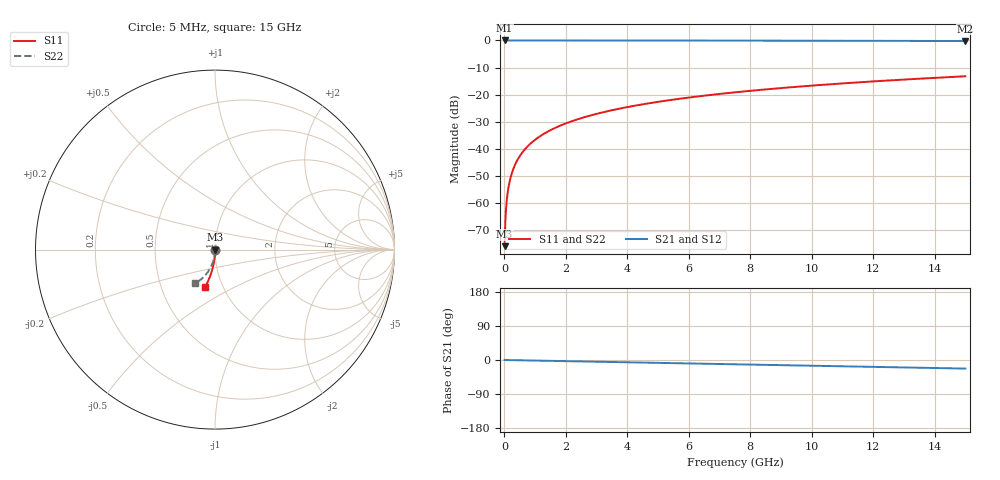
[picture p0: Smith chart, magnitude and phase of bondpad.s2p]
! Created Wed Jan 20 14:36:55 2021
# hz S ma R 50
! 2 Port Network Data from SP1.SP block
! freq  magS11  angS11  magS21  angS21  magS12  angS12  magS22  angS22
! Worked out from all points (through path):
!   3000 points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, 5 MHz to 15 GHz, reference 50 ohm
!   highest |S21| = 0.00 dB at 5 MHz (marker M1); lowest = -0.2 dB at 15 GHz (marker M2)
!   group delay of S21, straight-line fit = 4.19 ps
!   lowest |S11| = -75.9 dB at 5 MHz (marker M3), VSWR 1.00, Z = 50 - j0.00742 ohm
!   |S11| at or under -10 dB: start of sweep to end of sweep
!   |S22| runs from -75.9 to -13.2 dB; largest |S21 - S12| = 0
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5000000  0.0001606 -27.5  0.9999 -0.0  0.9999 -0.0  0.0001606 -27.5
4e7  0.0006096 -76.5  0.9999 -0.1  0.9999 -0.1  0.0006093 -76.5
8.5e7  0.001267 -83.6  0.9999 -0.1  0.9999 -0.1  0.001266 -83.7
1e8  0.001488 -84.6  0.9999 -0.2  0.9999 -0.2  0.001487 -84.7
1.3e8  0.00193 -85.9  0.9998 -0.2  0.9998 -0.2  0.001929 -86.0
1.7e8  0.00252 -86.9  0.9998 -0.3  0.9998 -0.3  0.002519 -87.1
2.3e8  0.003407 -87.8  0.9998 -0.3  0.9998 -0.3  0.003405 -88.0
3.1e8  0.004589 -88.5  0.9998 -0.5  0.9998 -0.5  0.004586 -88.8
4.1e8  0.006067 -89.0  0.9998 -0.6  0.9998 -0.6  0.006063 -89.4
5.25e8  0.007766 -89.5  0.9998 -0.8  0.9998 -0.8  0.007761 -90.0
6.7e8  0.009909 -89.8  0.9998 -1.0  0.9998 -1.0  0.009903 -90.5
8.4e8  0.01242 -90.2  0.9997 -1.3  0.9997 -1.3  0.01241 -91.0
1.04e9  0.01538 -90.5  0.9997 -1.6  0.9997 -1.6  0.01537 -91.5
1.265e9  0.0187 -90.8  0.9996 -1.9  0.9996 -1.9  0.01869 -92.1
1.815e9  0.02683 -91.5  0.9994 -2.7  0.9994 -2.7  0.0268 -93.3
2.505e9  0.03701 -92.3  0.9991 -3.8  0.9991 -3.8  0.03698 -94.8
3.61e9  0.05332 -93.5  0.9983 -5.5  0.9983 -5.5  0.05327 -97.1
5.005e9  0.07387 -95.0  0.9969 -7.6  0.9969 -7.6  0.07379 -99.9
7.505e9  0.1106 -97.6  0.9934 -11.3  0.9934 -11.3  0.1104 -104.9
1.0005e10  0.147 -100.1  0.9885 -15.1  0.9885 -15.1  0.1467 -110.0
1.2505e10  0.183 -102.6  0.9824 -18.9  0.9824 -18.9  0.1826 -115.0
1.5e10  0.2184 -105.1  0.975 -22.6  0.975 -22.6  0.2179 -120.0
